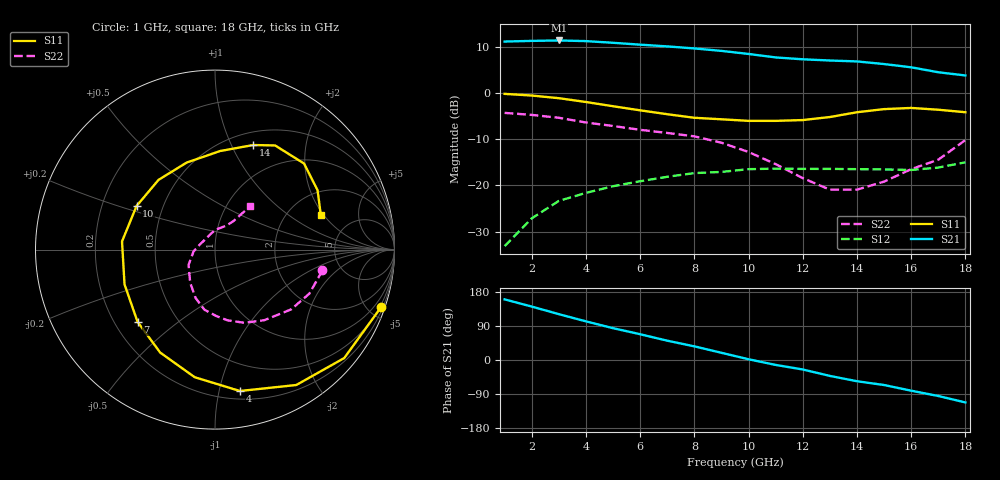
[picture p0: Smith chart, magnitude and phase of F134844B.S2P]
!ATF-13484
!S-PARAMETERS at Vds=4V  Id=40mA.  LAST UPDATED 07-22-92
# ghz s ma r 50
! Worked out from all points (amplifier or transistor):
!   18 points, 1 GHz to 18 GHz, reference 50 ohm
!   highest |S21| = 11.4 dB at 3 GHz (marker M1)
!   |S21| within 3 dB of that: start of sweep to 10.1 GHz
!   unconditionally stable (mu >= 1): 9.852 GHz to end of sweep
!   at 4 GHz: K = 0.58, MSG = 16.4 dB, |S12| = -21.6 dB
!   at 10 GHz: K = 1.01, MAG = 11.9 dB, |S12| = -16.5 dB
!   at 18 GHz: K = 1.11, MAG = 7.4 dB, |S12| = -15.0 dB
!   S11 on the Smith chart (normalised r, x): 1 GHz: 0.37, -5.95; 4 GHz: 0.26, -1.16; 7 GHz: 0.29, -0.36; 10 GHz: 0.35, +0.23; 14 GHz: 0.64, +1.21; 18 GHz: 3.00, +1.87
1  0.98 -19.0  3.61 160.0  0.022 74.0  0.61 -11.0
2  0.94 -40.0  3.67 141.0  0.044 65.0  0.58 -25.0
3  0.88 -59.0  3.71 121.0  0.068 48.0  0.54 -38.0
4  0.8 -80.0  3.65 102.0  0.083 38.0  0.48 -55.0
5  0.72 -99.0  3.5 84.0  0.098 27.0  0.44 -68.0
6  0.65 -118.0  3.34 68.0  0.111 19.0  0.4 -80.0
7  0.59 -137.0  3.2 51.0  0.124 7.0  0.37 -89.0
8  0.54 -159.0  3.04 36.0  0.136 0.0  0.34 -100.0
9  0.52 175.0  2.86 19.0  0.14 -12.0  0.29 -112.0
10  0.5 151.0  2.65 2.0  0.15 -21.0  0.23 -127.0
11  0.5 129.0  2.43 -13.0  0.152 -31.0  0.17 -150.0
12  0.51 108.0  2.32 -25.0  0.151 -40.0  0.12 -175.0
13  0.55 87.0  2.25 -42.0  0.151 -47.0  0.09 163.0
14  0.62 70.0  2.2 -56.0  0.15 -58.0  0.09 106.0
15  0.67 60.0  2.06 -66.0  0.149 -65.0  0.11 89.0
16  0.69 44.0  1.9 -81.0  0.147 -72.0  0.15 64.0
17  0.66 30.0  1.68 -95.0  0.156 -82.0  0.19 57.0
18  0.62 18.0  1.55 -112.0  0.178 -100.0  0.31 51.0
